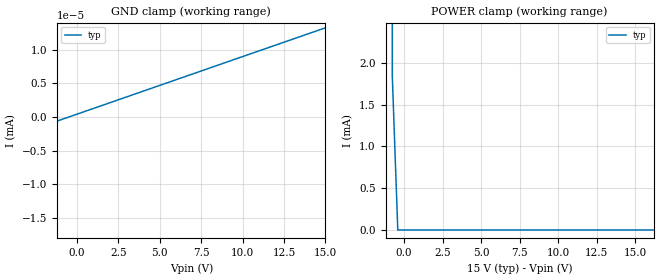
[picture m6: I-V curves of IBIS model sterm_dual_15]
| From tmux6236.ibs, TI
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| sterm_dual_15
[Model]   sterm_dual_15
Model_type   Terminator
|   typ   min   max
C_comp   4.014581e-11   NA   NA
[Voltage Range]   15   NA   NA
[Temperature Range]   27   NA   NA
[Power Clamp Reference]   15   NA   NA
[GND Clamp Reference]   0   NA   NA
[GND Clamp]
|   Voltage   I(typ)   I(min)   I(max)
-20V      -7.108A    NA         NA
-15.4V    -362.8nA   NA         NA
-15.05V   -12.47nA   NA         NA
15V       13.28nA    NA         NA
[POWER Clamp]
|   Voltage   I(typ)   I(min)   I(max)
-5V       7.349A     NA         NA
-1.111V   157.6mA    NA         NA
-757.6mV  1.832mA    NA         NA
-404mV    417.9nA    NA         NA
30V       -12.41nA   NA         NA
